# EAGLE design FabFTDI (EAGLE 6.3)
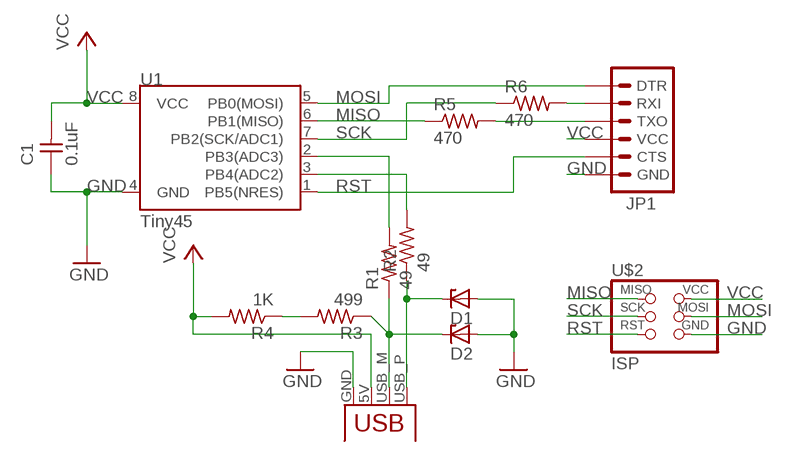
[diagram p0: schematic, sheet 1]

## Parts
C1  0.1uF  UNPOLARIZED_CAPACITOR1206  [1206]
D1  ZENER_DIODESOD123  [SOD123]
D2  ZENER_DIODESOD123  [SOD123]
JP1  FTDI_CONNECTORSMD  [1X06-SMD]
JP2  USBPCB  [USB-A-PCB]
R1  49  RESISTOR1206  [1206]
R2  49  RESISTOR1206  [1206]
R3  499  RESISTOR1206  [1206]
R4  1K  RESISTOR1206  [1206]
R5  470  RESISTOR1206  [1206]
R6  470  RESISTOR1206  [1206]
U1  Tiny45  ATTINY45TINY45-20-SMT  [SO08-EIAJ]
U$2  ISP  AVRISPSMD  [2X03SMD]

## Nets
GND: C1.1 D1.ANODE D2.ANODE JP1.6(GND) JP2.GND U1.4(GND) U$2.6(GND)
MISO: R5.1 U1.6(PB1(MISO)) U$2.1(MISO)
MOSI: JP1.1(DTR) U1.5(PB0(MOSI)) U$2.4(MOSI)
N$1: D1.CATHODE JP2.USB_P(D+) R2.1
N$2: D2.CATHODE JP2.USB_M(D-) R1.1 R3.1
N$3: R1.2 U1.2(PB3(ADC3))
N$4: R2.2 U1.3(PB4(ADC2))
N$5: R3.2 R4.1
N$7: JP1.2(RXI) R6.2
N$8: JP1.3(TXO) R5.2
RST: JP1.5(CTS) U1.1(PB5(NRES)) U$2.5(RST)
SCK: R6.1 U1.7(PB2(SCK/ADC1)) U$2.3(SCK)
VCC: C1.2 JP1.4(VCC) JP2.5V(VBUS) R4.2 U1.8(VCC) U$2.2(VCC)

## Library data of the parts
C1 = fabPatil:UNPOLARIZED_CAPACITOR: unpolarized_capacitor
D1 D2 = fabPatil:ZENER_DIODE: zener diode
JP1 = fabPatil:FTDI_CONNECTOR: FTDI connector smd
JP2 = fabPatil:USB: USB Connectors USB-B-PTH is fully proven SKU : PRT-00139/CONN-08278 USB-miniB is fully proven SKU : PRT-00587 USB-A-PCB is untested. USB-A-H is throughly reviewed, but untested. Spark Fun Electronics SKU : PRT-00437 USB-B-SMT is throughly reviewed, but untested. Needs silkscreen touching up.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
R1-R6 = fabPatil:RESISTOR
U1 = fabPatil:ATTINY45: Atmel 8-pin 2/4/8kB flash uC; PROD_ID: IC-08922; VALUE: Tiny45-20-SMT
U$2 = fabPatil:AVRISP

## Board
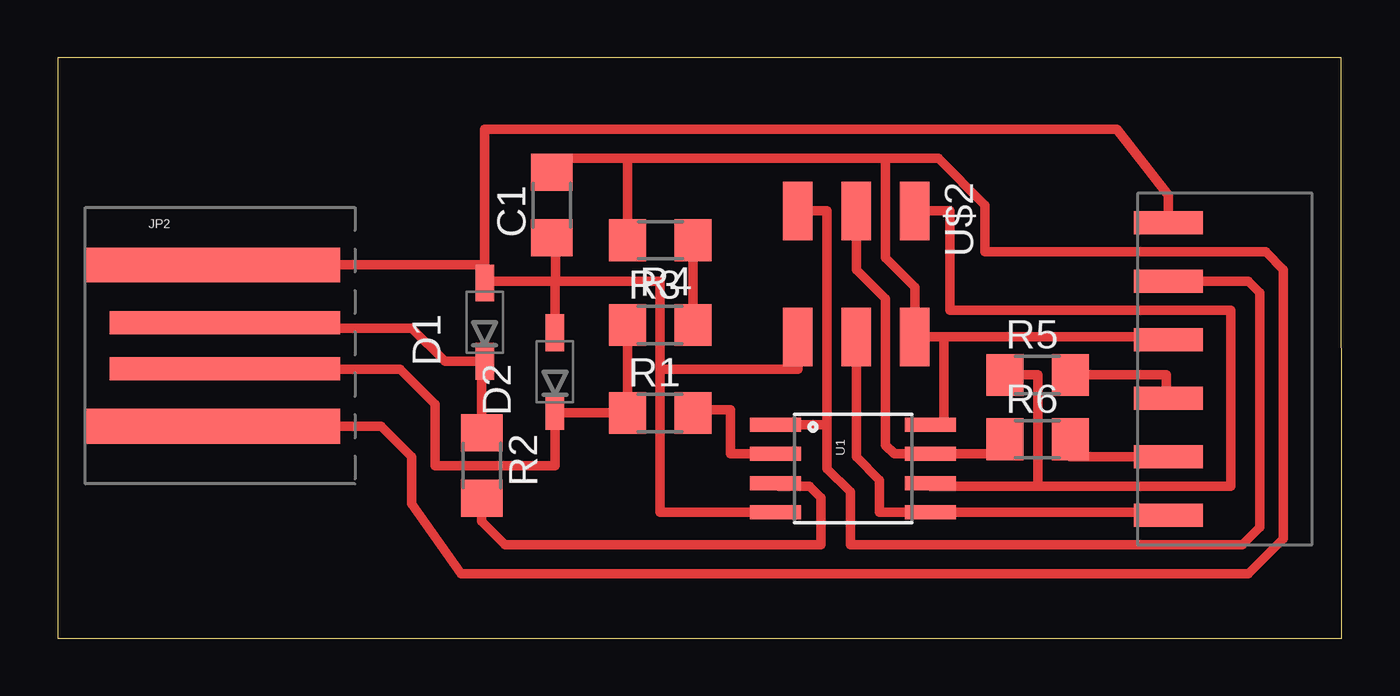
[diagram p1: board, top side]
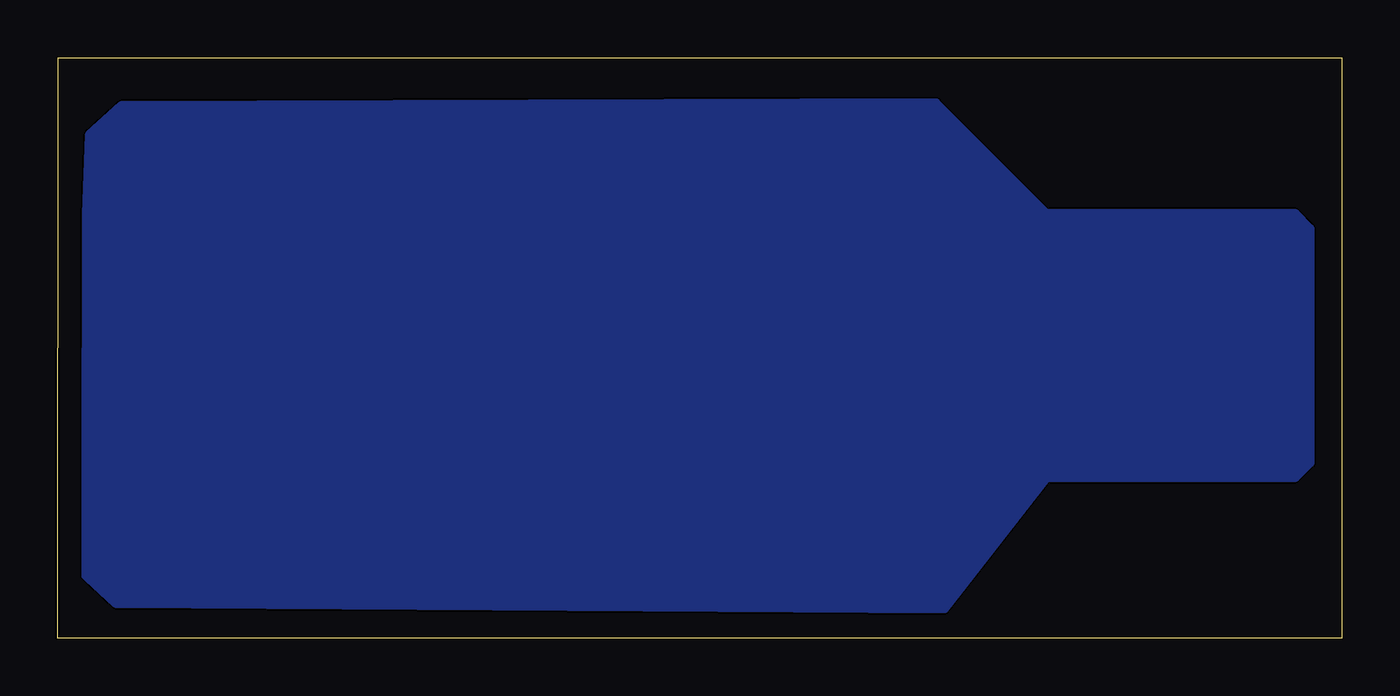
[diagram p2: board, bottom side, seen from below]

Size 55.75 x 25.2 mm. Coordinates in mm from the lower left corner, seen from the top.
Outline: 0,0 55.75,0 55.73,25.2 0,25.2 0,0
Copper layers (1*16): Top 0.035mm / dielectric 1.5mm / Bottom 0.035mm
Design rules "default": minimum track width 10mil, minimum drill 24mil, track to track 8mil, track to pad 8mil, pad to pad 8mil, via to via 8mil, smd to smd 8mil, copper to edge 40mil, drill to drill 8mil, minimum pad ring 10mil, minimum via ring 8mil, stop-mask expansion 4mil, vias tented up to drill 0mil, thermal gap 10mil

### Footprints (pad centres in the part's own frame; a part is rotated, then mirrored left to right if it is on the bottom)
1206 = smd 1.6 x 1.803: 1 -1.422,0; 2 1.422,0
SOD123 = smd 1.6 x 0.8: ANODE 1.7,0; CATHODE -1.7,0
1X06-SMD = smd 1 x 3: 1 -6.35,5; 2 -3.81,5; 3 -1.27,5; 4 1.27,5; 5 3.81,5; 6 6.35,5
USB-A-PCB = smd 11 x 1.5: 5V 1.55,-3.5; GND 1.55,3.5 | smd 10 x 1: USB_M 2.05,-1; USB_P 2.05,1
SO08-EIAJ = smd 0.61 x 2.21: 1 -1.905,-3.378; 2 -0.635,-3.378; 3 0.635,-3.378; 4 1.905,-3.378; 5 1.905,3.353; 6 0.635,3.353; 7 -0.635,3.353; 8 -1.905,3.353
2X03SMD = smd 2.54 x 1.27: 1 -2.54,2.54; 2 2.92,2.54; 3 -2.54,0; 4 2.92,0; 5 -2.54,-2.54; 6 2.92,-2.54

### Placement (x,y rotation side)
C1  21.46,18.8 90 top
D1  18.54,13.72 90 top
D2  21.59,11.56 90 top
JP1  53.21,11.68 90 top
JP2  5.21,12.7 0 top
R1  26.16,9.78 0 top
R2  18.41,7.49 270 top
R3  26.16,13.59 0 top
R4  26.16,17.27 180 top
R5  42.54,11.43 0 top
R6  42.54,8.64 0 top
U1  34.54,7.37 270 top
U$2  34.67,16 270 top

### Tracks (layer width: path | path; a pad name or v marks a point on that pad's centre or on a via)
GND
  Top 0.406: 48.39,18.03 JP1.6 48.21,19.22 45.97,22.1 18.54,22.1 18.54,16.26 | U$2.6 32.13,11.68 26.16,11.68 | 26.16,11.68 26.16,15.49 21.59,15.49 | D2.ANODE 21.59,15.49 | 21.59,15.49 18.37,15.49 arc90 D1.ANODE 18.54,16.26 | U1.4 26.16,5.46 26.16,11.68 | 21.59,15.49 21.62,15.52 21.62,17.37 C1.1 | JP2.GND 18.49,16.2 18.54,16.26
MISO
  Top 0.406: U$2.1 38.73,18.54 38.73,14.22 50.93,14.22 50.93,6.6 42.54,6.6 | 42.54,6.6 42.54,11.43 R5.1 | 42.54,6.6 37.9,6.6 U1.6
MOSI
  Top 0.406: JP1.1 48.21,5.46 U1.5 35.69,5.46 35.69,6.86 34.67,7.87 U$2.4
N$1
  Top 0.406: R2.1 18.41,11.89 arc90 D1.CATHODE 16.81,12.02 15.37,13.46 9.81,13.46 JP2.USB_P
N$2
  Top 0.406: R1.1 24.77,9.78 | R1.1 R3.1 | R1.1 21.67,9.78 D2.CATHODE 21.59,7.49 16.38,7.49 16.38,10.16 14.86,11.68 9.59,11.68 JP2.USB_M
N$3
  Top 0.406: U1.2 29.21,8 29.21,9.91 27.33,9.91 R1.2
N$4
  Top 0.406: U1.3 31.29,6.6 32.64,6.6 33.15,6.1 33.15,4.06 19.43,4.06 18.41,5.08 R2.2
N$5
  Top 0.406: R3.2 R4.1
N$6
  pour Bottom (no thermals): 1.4,17.78 2.03,18.41 12.83,18.41 17.65,23.24 52.96,23.11 54.36,21.84 arc-3 54.74,2.92 53.21,1.52 17.27,1.27 12.83,6.99 2.03,6.99 1.4,7.62
N$7
  Top 0.406: JP1.2 43.97,7.87 R6.2
N$8
  Top 0.406: JP1.3 48.13,10.41 48.13,11.43 R5.2
RST
  Top 0.406: 30.35,9.27 U1.1 33.4,9.27 | 33.4,9.27 33.4,18.54 U$2.5 | JP1.5 51.69,15.49 52.2,14.99 52.2,4.83 51.43,4.06 34.42,4.06 34.42,6.35 33.4,7.37 33.4,9.27
SCK
  Top 0.406: 34.42,18.54 U$2.3 34.67,16 35.94,14.73 35.94,8.38 36.32,8 U1.7 41.12,8 R6.1
VCC
  Top 0.406: 38.48,13.08 U$2.2 37.21,15.24 35.94,16.51 35.94,20.83 | 38.48,13.08 48.21,13.08 JP1.4 | U1.8 38.48,9.27 38.48,13.08 | 35.94,20.83 24.74,20.83 | 24.74,20.83 R4.2 | 24.74,20.83 21.46,20.83 C1.2 | 35.94,20.83 38.23,20.83 40.26,18.8 40.26,16.76 52.45,16.76 53.21,16 53.21,4.32 51.69,2.79 17.53,2.79 15.37,5.84 15.37,7.87 14.04,9.2 JP2.5V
